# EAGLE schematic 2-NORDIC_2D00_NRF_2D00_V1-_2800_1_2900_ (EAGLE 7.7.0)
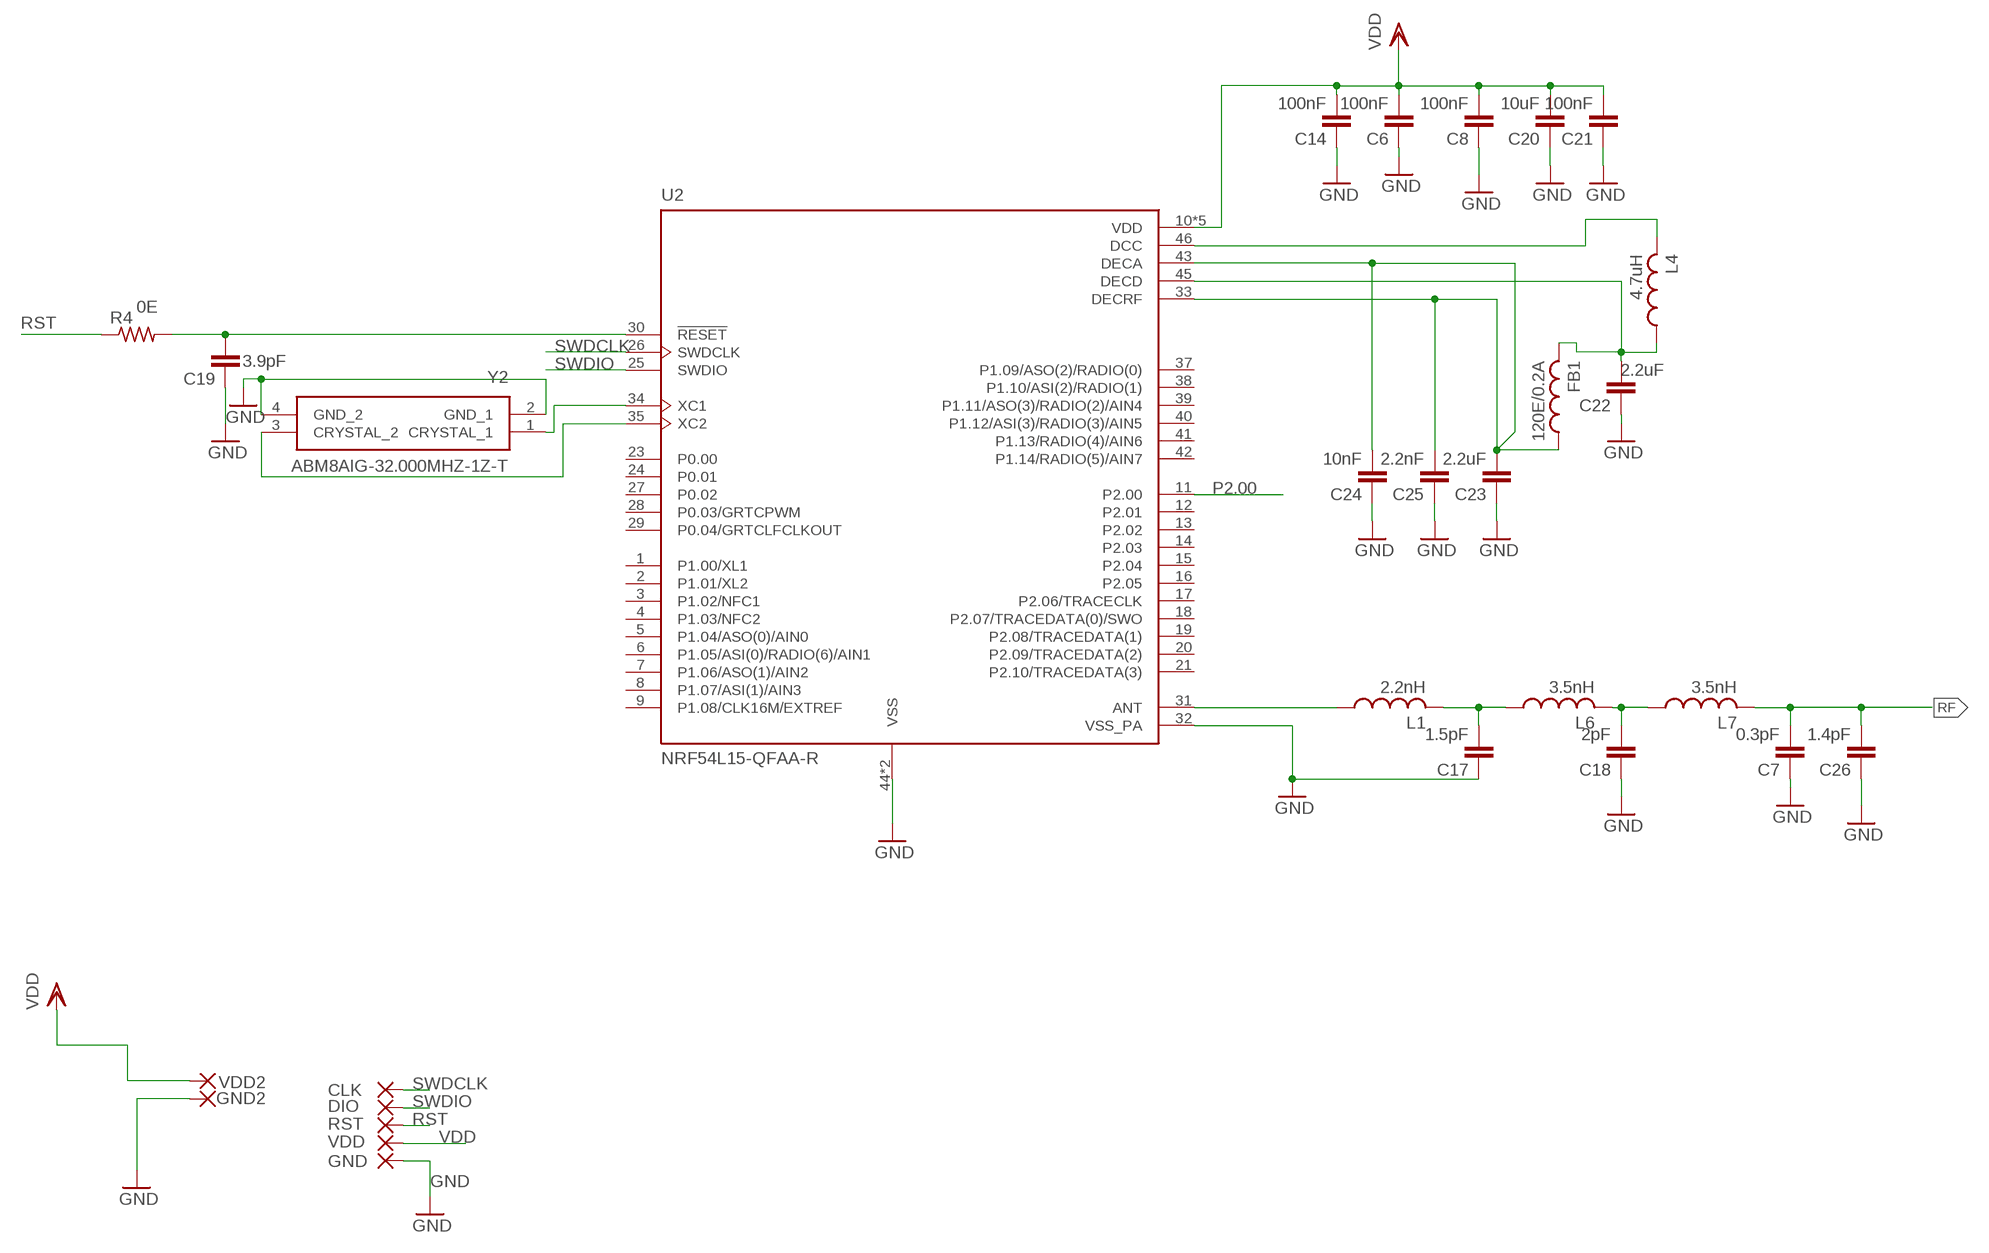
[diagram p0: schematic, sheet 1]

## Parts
C6  100nF  C-EUC0201  [C0201]
C7  0.3pF  C-EUC0201  [C0201]
C8  100nF  C-EUC0201  [C0201]
C14  100nF  C-EUC0201  [C0201]
C17  1.5pF  C-EUC0201  [C0201]
C18  2pF  C-EUC0201  [C0201]
C19  3.9pF  C-EUC0201  [C0201]
C20  10uF  C-EUC0402  [C0402]
C21  100nF  C-EUC0201  [C0201]
C22  2.2uF  C-EUC0201  [C0201]
C23  2.2uF  C-EUC0201  [C0201]
C24  10nF  C-EUC0201  [C0201]
C25  2.2nF  C-EUC0201  [C0201]
C26  1.4pF  C-EUC0201  [C0201]
CLK  SMD2  [SMD2]
DIO  SMD2  [SMD2]
FB1  120E/0.2A  L-USL0201  [L0201]
GND  SMD2  [SMD2]
GND2  SMD2  [SMD2]
L1  2.2nH  L-USL0201  [L0201]
L4  4.7uH  L-US  [INDC1608X100N]
L6  3.5nH  L-USL0201  [L0201]
L7  3.5nH  L-USL0201  [L0201]
R4  0E  R-US_R0201  [R0201]
RST  SMD2  [SMD2]
U2  NRF54L15-QFAA-R  [QFN40P600X600X90-49N]
VDD  SMD2  [SMD2]
VDD2  SMD2  [SMD2]
Y2  ABM8AIG-32.000MHZ-1Z-T  [ABM8AIG12000MHZ12D2ZT]

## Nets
GND: C6.1 C7.1 C8.1 C14.1 C17.1 C18.1 C19.1 C20.1 C21.1 C22.1 C23.1 C24.1 C25.1 C26.1 GND2.1(P) GND.1(P) U2.32(VSS_PA) U2.44(VSS) U2.49(VSS) Y2.2(GND_1) Y2.4(GND_2)
N$3: L1.1 U2.31(ANT)
N$12: U2.34(XC1) Y2.1(CRYSTAL_1)
N$14: U2.35(XC2) Y2.3(CRYSTAL_2)
N$16: C19.2 R4.2 U2.30(!RESET)
N$18: L4.2 U2.46(DCC)
N$19: C22.2 FB1.2 L4.1 U2.45(DECD)
N$20: C18.2 L6.2 L7.1
N$21: C23.2 C24.2 C25.2 FB1.1 U2.33(DECRF) U2.43(DECA)
N$22: C17.2 L1.2 L6.1
P2.00: U2.11(P2.00)
RF: C7.2 C26.2 L7.2
RST: R4.1 RST.1(P)
SWDCLK: CLK.1(P) U2.26(SWDCLK)
SWDIO: DIO.1(P) U2.25(SWDIO)
VDD: C6.2 C8.2 C14.2 C20.2 C21.2 U2.10(VDD) U2.22(VDD) U2.36(VDD) U2.47(VDD) U2.48(VDD) VDD2.1(P) VDD.1(P)
Unconnected: U2.1(P1.00/XL1) U2.2(P1.01/XL2) U2.3(P1.02/NFC1) U2.4(P1.03/NFC2) U2.5(P1.04/ASO(0)/AIN0) U2.6(P1.05/ASI(0)/RADIO(6)/AIN1) U2.7(P1.06/ASO(1)/AIN2) U2.8(P1.07/ASI(1)/AIN3) U2.9(P1.08/CLK16M/EXTREF) U2.12(P2.01) U2.13(P2.02) U2.14(P2.03) U2.15(P2.04) U2.16(P2.05) U2.17(P2.06/TRACECLK) U2.18(P2.07/TRACEDATA(0)/SWO) U2.19(P2.08/TRACEDATA(1)) U2.20(P2.09/TRACEDATA(2)) U2.21(P2.10/TRACEDATA(3)) U2.23(P0.00) U2.24(P0.01) U2.27(P0.02) U2.28(P0.03/GRTCPWM) U2.29(P0.04/GRTCLFCLKOUT) U2.37(P1.09/ASO(2)/RADIO(0)) U2.38(P1.10/ASI(2)/RADIO(1)) U2.39(P1.11/ASO(3)/RADIO(2)/AIN4) U2.40(P1.12/ASI(3)/RADIO(3)/AIN5) U2.41(P1.13/RADIO(4)/AIN6) U2.42(P1.14/RADIO(5)/AIN7)

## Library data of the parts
C6-C8 C14 C17-C26 = rcl:C-EU: CAPACITOR, European symbol
CLK DIO GND GND2 RST VDD VDD2 = wirepad:SMD2: SMD PAD
FB1 L1 L4 L6 L7 = rcl:L-US: INDUCTOR, American symbol
R4 = rcl:R-US_: 55mmx 10mm
U2 = NRF54L15-QFAA-R:NRF54L15-QFAA-R; MANUFACTURER: Nordic; MAXIMUM_PACKAGE_HEIGHT: 0.9mm; PARTREV: 0.8; STANDARD: IPC-7351B
Y2 = ABM8AIG-32.000MHZ-1Z-T:ABM8AIG-32.000MHZ-1Z-T: Crystals 18pF 32MHz 10ppm AEC-Q200 -40C +125C Source: Datasheet; DESCRIPTION: Crystals 18pF 32MHz 10ppm AEC-Q200 -40C +125C; HEIGHT: 0.8mm; MANUFACTURER_NAME: ABRACON; MANUFACTURER_PART_NUMBER: ABM8AIG-32.000MHZ-1Z-T; MOUSER_PART_NUMBER: 815-M8AIG-32-1ZT; MOUSER_PRICE-STOCK: https://www.mouser.com/Search/Refine.aspx?Keyword=815-M8AIG-32-1ZT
